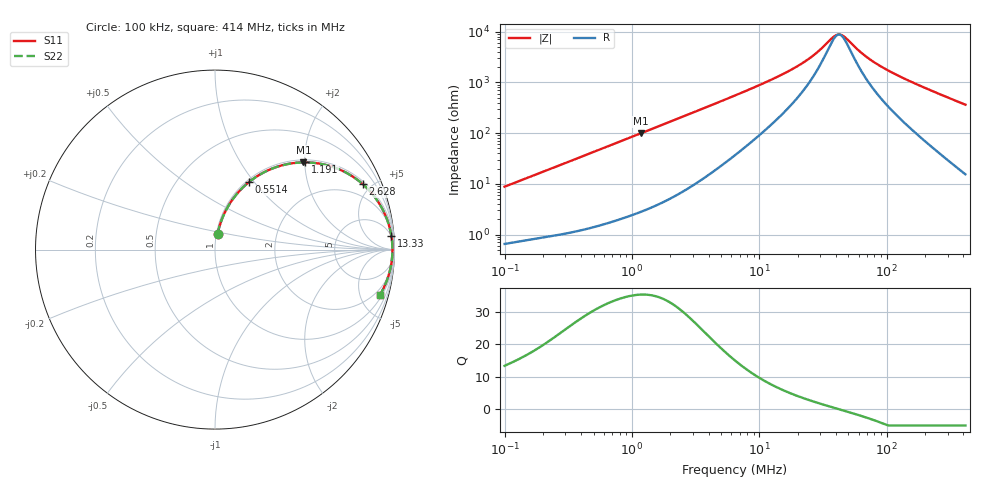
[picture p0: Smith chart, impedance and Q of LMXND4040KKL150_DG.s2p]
! LMXND4040KKL150_DG  S-PARAMETER MODEL  ( General Type )
! Model Generated by TAIYO YUDEN Corporation (http://www.ty-top.com)
! Version 1.0
! TAIYO YUDEN Control No. 191023NI43SB-FBB
! Copyright(c) 2019 TAIYO YUDEN CO.,LTD. All Rights Reserved.
! Product Description (link to TY-COMPAS)
! https://ds.yuden.co.jp/TYCOMPAS/or/detail?pn=LMXND4040KKL150MDG&u=M
! Products Name : Inductors
! Characteristics :
!  Inductance : 15 uH , SRF(min) : 24 MHz , DC Resistance(max) : 0.516 Ohm
!  Rated Current : Saturation :540 mA , Temp Rise : 600 mA
!  Case Size : 4.0 x 4.0 / 0.157 x 0.157 [mm/inch] , Thickness : 1 / 0.039 [mm/inch]
!  (Conditions: Temperature = 25 degC , DC Bias Current/Voltage = 0A / 0V)
! External Node Assignments :
!  1  o---GGG---o  2
! GND o---------o GND
! Frequency Range : 0.1MHz  -  413.982163MHz  [ 402 STEP ]
# MHz S RI R 50
! Freq[MHz].  S11 Real  S11 Imag  S21 Real  S21 Imag  S12 Real  S12 Imag  S22 Real  S22 Imag
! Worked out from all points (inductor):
!   401 points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, 100 kHz to 414 MHz, reference 50 ohm
!   read as one part in series: L = 13.8 uH near 104.3 kHz
!   highest Q = 35.3 at 1.167 MHz (marker M1), where L = 13.4 uH
!   self-resonance near 42.14 MHz
!   S11 on the Smith chart (normalised r, x): 100 kHz: 1.01, +0.17; 551.4 kHz: 1.03, +0.94; 1.191 MHz: 1.06, +2.01; 2.628 MHz: 1.15, +4.42; 13.33 MHz: 4, +24; 414 MHz: 1.31, -7.25
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0.1  0.0139 0.0857  0.9861 -0.0857  0.9861 -0.0857  0.0139 0.0857
0.202975  0.0376 0.1667  0.9624 -0.1667  0.9624 -0.1667  0.0376 0.1667
0.403501  0.1143 0.301  0.8857 -0.301  0.8857 -0.301  0.1143 0.301
0.551418  0.1877 0.3749  0.8123 -0.3749  0.8123 -0.3749  0.1877 0.3749
0.836239  0.338 0.4587  0.662 -0.4587  0.662 -0.4587  0.338 0.4587
1.166835  0.4923 0.486  0.5077 -0.486  0.5077 -0.486  0.4923 0.486
1.191385  0.5023 0.4861  0.4977 -0.4861  0.4977 -0.4861  0.5023 0.4861
1.628129  0.6486 0.4632  0.3514 -0.4632  0.3514 -0.4632  0.6486 0.4632
2.628242  0.8222 0.3657  0.1778 -0.3657  0.1778 -0.3657  0.8222 0.3657
3.98579  0.9091 0.2661  0.0909 -0.2661  0.0909 -0.2661  0.9091 0.2661
6.434145  0.9574 0.1713  0.0426 -0.1713  0.0426 -0.1713  0.9574 0.1713
13.3345  0.9824 0.0782  0.0176 -0.0782  0.0176 -0.0782  0.9824 0.0782
19.39728  0.9864 0.0473  0.0136 -0.0473  0.0136 -0.0473  0.9864 0.0473
25.96183  0.9879 0.0279  0.0121 -0.0279  0.0121 -0.0279  0.9879 0.0279
37.76586  0.9887 0.00608  0.0113 -0.00608  0.0113 -0.00608  0.9887 0.00608
40.20007  0.9887 0.0026  0.0113 -0.0026  0.0113 -0.0026  0.9887 0.0026
42.79117  0.9888 -0.000855  0.0112 0.000855  0.0112 0.000855  0.9888 -0.000855
47.48609  0.9887 -0.00664  0.0113 0.00664  0.0113 0.00664  0.9887 -0.00664
70.52986  0.9879 -0.0298  0.0121 0.0298  0.0121 0.0298  0.9879 -0.0298
104.7562  0.9854 -0.0575  0.0146 0.0575  0.0146 0.0575  0.9854 -0.0575
191.6068  0.9744 -0.1181  0.0256 0.1181  0.0256 0.1181  0.9744 -0.1181
413.9822  0.9202 -0.2505  0.0798 0.2505  0.0798 0.2505  0.9202 -0.2505
